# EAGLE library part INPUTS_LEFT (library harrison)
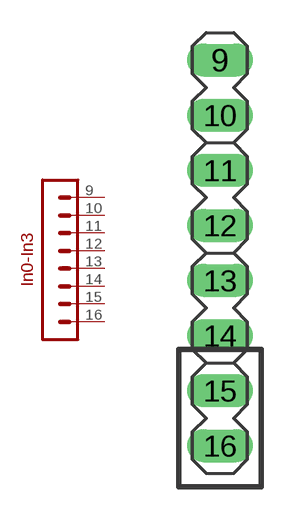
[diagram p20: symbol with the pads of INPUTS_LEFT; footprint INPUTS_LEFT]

Designator prefix -

## INPUTS_LEFT  [INPUTS_LEFT]
9  P$8  pas
10  P$7  pas
11  P$6  pas
12  P$5  pas
13  P$4  pas
14  P$3  pas
15  P$2  pas
16  P$1  pas

## Footprint INPUTS_LEFT (pad centres in mm)
drill 1.016 long: 9 0,-0.635; 10 0,-3.175; 11 0,-5.715; 12 0,-8.255; 13 0,-10.795; 14 0,-13.335; 15 0,-15.875; 16 0,-18.415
